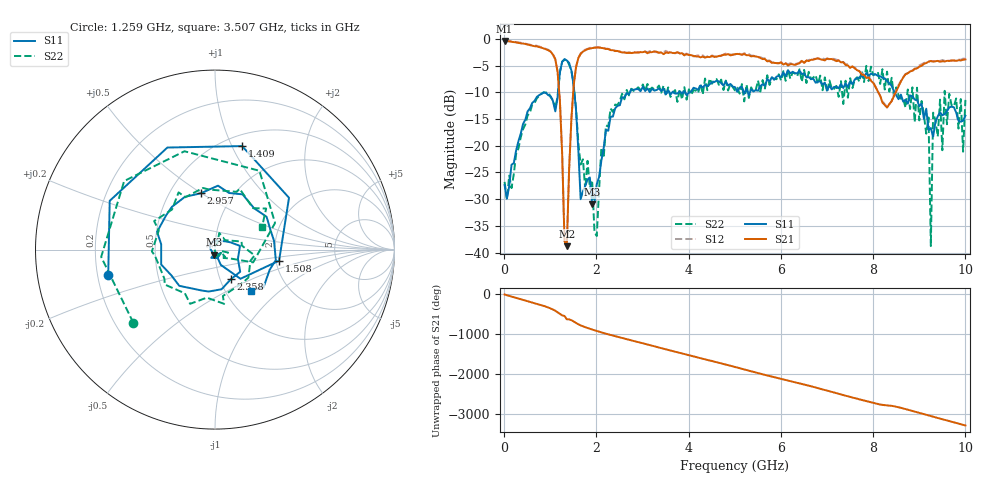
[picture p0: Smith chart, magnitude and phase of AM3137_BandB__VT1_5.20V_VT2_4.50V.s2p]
! Date/Time: Tue, Nov 13, 2018 4:52 PM
! Network Analyzer: Agilent Technologies E8364B Rev: A.07.50.67
! Sweep from 0.010 to 10.000 GHz, 201 Points, Sweep Type: LIN
! Power Supply: 5.201 V, 0.002 A
# Hz S DB R 50
!freq MagS11 AngS11 MagS21 AngS21 MagS12 AngS12 MagS22 AngS22
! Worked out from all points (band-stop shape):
!   201 points, 10 MHz to 10 GHz, reference 50 ohm
!   highest |S21| = -0.39 dB at 10 MHz (marker M1); lowest = -38.8 dB at 1.359 GHz (marker M2)
!   |S21| within 3 dB of the highest: start of sweep to 1.084 GHz; 1.622 GHz to 4.235 GHz (2.613 GHz wide, 89.2 % of centre)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
!   lowest |S11| = -31.0 dB at 1.908 GHz (marker M3), VSWR 1.06, Z = 49.3 - j2.71 ohm
!   |S11| at or under -10 dB: start of sweep to 1.169 GHz; 1.522 GHz to 2.729 GHz (1.207 GHz wide, 56.8 % of centre); 8.463 GHz to end of sweep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
!   |S22| runs from -38.8 to -3.9 dB; largest |S21 - S12| = 0.037
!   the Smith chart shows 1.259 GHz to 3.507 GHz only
!   S11 on the Smith chart (normalised r, x): 1.259 GHz: 0.24, -0.11; 1.409 GHz: 0.61, +1.10; 1.508 GHz: 2.08, -0.29; 2.358 GHz: 1.12, -0.39; 2.957 GHz: 0.71, +0.50; 3.507 GHz: 1.31, -0.66
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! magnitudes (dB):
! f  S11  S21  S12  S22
! 10 MHz  -27.4  -0.4  -0.4  -26.8
! 1.059 GHz  -11.6  -3.0  -2.9  -11.4
! 1.259 GHz  -4.3  -21.8  -21.6  -4.3
! 1.359 GHz  -4.0  -38.8  -38.8  -4.0
! 1.409 GHz  -4.5  -24.4  -24.4  -4.8
! 1.508 GHz  -8.8  -8.7  -8.6  -8.7
! 1.708 GHz  -28.6  -2.4  -2.3  -22.5
! 1.908 GHz  -31.0  -1.7  -1.7  -26.5
! 2.008 GHz  -27.2  -1.6  -1.6  -36.9
! 2.108 GHz  -22.8  -1.7  -1.6  -20.4
! 2.358 GHz  -14.5  -2.1  -2.1  -13.7
! 2.957 GHz  -9.8  -2.5  -2.5  -9.6
! 3.357 GHz  -9.3  -2.6  -2.6  -8.7
! 3.507 GHz  -10.4  -2.5  -2.2  -10.7
! 5.005 GHz  -9.0  -2.9  -2.9  -9.7
! 6.703 GHz  -7.5  -3.9  -3.8  -7.2
! 8.352 GHz  -8.3  -12.2  -12.3  -9.9
! 9.201 GHz  -17.0  -4.3  -4.3  -14.7
! 9.251 GHz  -16.7  -4.2  -4.1  -38.8
! 9.301 GHz  -18.3  -4.2  -4.2  -13.8
! 9.95 GHz  -15.3  -3.9  -3.7  -21.1
! 10 GHz  -14.4  -3.9  -3.7  -11.4
